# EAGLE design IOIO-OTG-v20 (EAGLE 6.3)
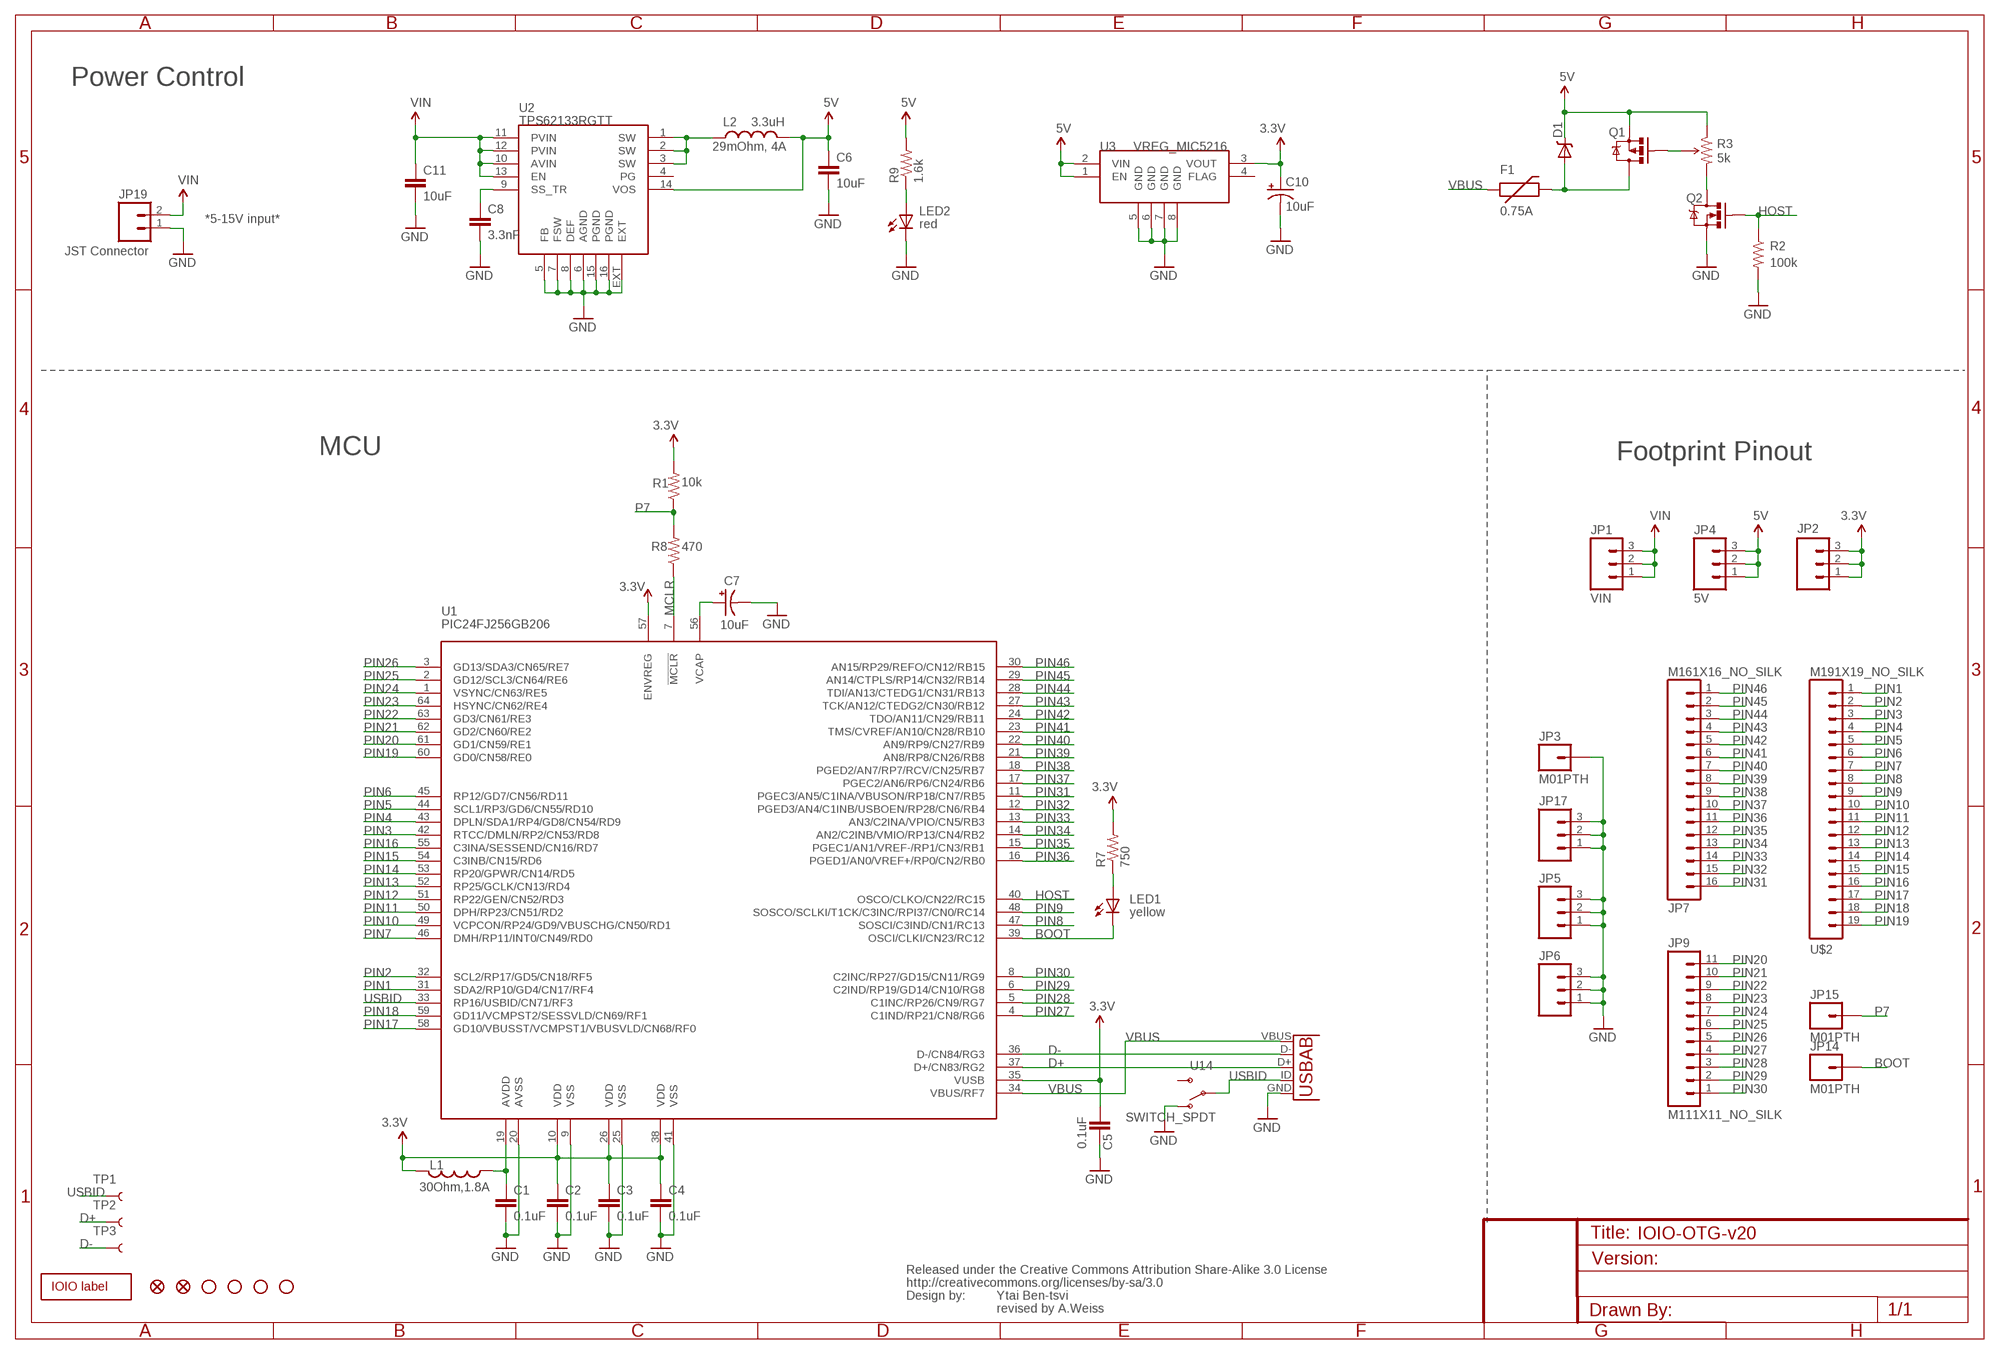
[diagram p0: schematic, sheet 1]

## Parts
C1  0.1uF  CAP0402-CAP  [0402-CAP]
C2  0.1uF  CAP0402-CAP  [0402-CAP]
C3  0.1uF  CAP0402-CAP  [0402-CAP]
C4  0.1uF  CAP0402-CAP  [0402-CAP]
C5  0.1uF  CAP0402-CAP  [0402-CAP]
C6  10uF  CAP0805  [0805]
C7  10uF  CAP_POL1206  [EIA3216]
C8  3.3nF  CAP0402-CAP  [0402-CAP]
C10  10uF  CAP_POL1206  [EIA3216]
C11  10uF  CAP1210  [1210]
D1  B340A  DIODE-SCHOTTKY_  [SMA-DIODE]
F1  PTCSMD  [PTC-1206]
JP1  VIN  M03PTH  [1X03]
JP2  M03PTH  [1X03]
JP3  M01PTH  [1X01]
JP4  5V  M03PTH  [1X03]
JP5  M03PTH  [1X03]
JP6  M03PTH  [1X03]
JP7  M161X16_NO_SILK  [1X16_NO_SILK]
JP8  FIDUCIALUFIDUCIAL  [MICRO-FIDUCIAL]
JP9  M111X11_NO_SILK  [1X11_NO_SILK]
JP10  STAND-OFF  [STAND-OFF]
JP11  STAND-OFF  [STAND-OFF]
JP12  STAND-OFF  [STAND-OFF]
JP13  STAND-OFF  [STAND-OFF]
JP14  M01PTH  [1X01]
JP15  M01PTH  [1X01]
JP16  FIDUCIALUFIDUCIAL  [MICRO-FIDUCIAL]
JP17  M03PTH  [1X03]
JP19  JST Connector  M02-JST-2MM-SMT  [JST-2-SMD]
L1  30Ohm,1.8A  INDUCTOR0402  [C0402]
L2  VLC5045T-3R3N  INDUCTORCR54  [CR54]
LED1  LY L29K-J1K2-26-Z  LED0603  [LED-0603]
LED2  LS L29K-G1J2-1-Z  LED0603  [LED-0603]
Q1  IRLML2244  MOSFET-PCHANNELSMD  [SOT23-3]
Q2  2N7002PW  MOSFET-NCHANNELSOT323  [SOT323]
R1  10k  RESISTOR0402-RES  [0402-RES]
R2  100k  RESISTOR0402-RES  [0402-RES]
R3  TS53YL502MR10  TRIMPOTTRIMPOT-5MM  [TRIMPOT-5MM]
R7  750  RESISTOR0402-RES  [0402-RES]
R8  470  RESISTOR0402-RES  [0402-RES]
R9  1.6k  RESISTOR0402-RES  [0402-RES]
TP1  TEST-POINT3  [PAD.03X.03]
TP2  TEST-POINT3  [PAD.03X.03]
TP3  TEST-POINT3  [PAD.03X.03]
U1  PIC24FJ256GB206  PIC24FXXXDAX06  [PIC24FXXX_TQFP64]
U2  TPS62133RGTT  TPS6214X  [QFN16-3X3MM]
U3  VREG_MIC5216  [MSOP8]
U14  SWITCH_SPDT  [KPS-1290]
U$1  CREATIVE_COMMONS  [CREATIVE_COMMONS]
U$2  M191X19_NO_SILK  [1X19_NO_SILK]
U$3  10104111-0001LF  USB_AB  [USB-AB-MICRO-SMD]
U$6  IOIO-OTG  [IOIO-OTG-COPPER-EXPOSED]

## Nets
3.3V: C2.1 C3.1 C4.1 C5.1 C10.A(+) JP2.1 JP2.2 JP2.3 L1.2 R1.2 R7.2 U1.10(VDD) U1.26(VDD) U1.35(VUSB) U1.38(VDD) U1.57(ENVREG) U3.3(VOUT)
5V: C6.1 D1.C JP4.1 JP4.2 JP4.3 L2.P$2 Q1.2(S) R3.A(CCW) R9.2 U2.14(VOS) U3.1(EN) U3.2(VIN)
BOOT: JP14.1 LED1.C U1.39(OSCI/CLKI/CN23/RC12)
D+: TP2.P$1 U1.37(D+/CN83/RG2) U$3.D+
D-: TP3.P$1 U1.36(D-/CN84/RG3) U$3.D-
GND: C1.2 C2.2 C3.2 C4.2 C5.2 C6.2 C7.C(-) C8.2 C10.C(-) C11.2 JP3.1 JP5.1 JP5.2 JP5.3 JP6.1 JP6.2 JP6.3 JP17.1 JP17.2 JP17.3 JP19.1 LED2.C Q2.2(S) R2.2 U1.9(VSS) U1.20(AVSS) U1.25(VSS) U1.41(VSS) U2.5(FB) U2.6(AGND) U2.7(FSW) U2.8(DEF) U2.15(PGND) U2.16(PGND) U2.EXT U3.5(GND) U3.6(GND) U3.7(GND) U3.8(GND) U14.O U$3.GND
HOST: Q2.1(G) R2.1 U1.40(OSCO/CLKO/CN22/RC15)
MCLR: R8.1 U1.7(!MCLR)
N$1: Q1.1(G) R3.B(WIPER)
N$2: LED1.A R7.1
N$3: LED2.A R9.1
N$4: D1.A F1.2 Q1.3(D)
N$5: C7.A(+) U1.56(VCAP)
N$6: L2.P$1 U2.1(SW) U2.2(SW) U2.3(SW)
N$7: C8.1 U2.9(SS_TR)
N$8: Q2.3(D) R3.C(CW)
N$9: C1.1 L1.1 U1.19(AVDD)
P7: JP15.1 R1.1 R8.2
PIN1: U1.31(SDA2/RP10/GD4/CN17/RF4) U$2.1
PIN2: U1.32(SCL2/RP17/GD5/CN18/RF5) U$2.2
PIN3: U1.42(RTCC/DMLN/RP2/CN53/RD8) U$2.3
PIN4: U1.43(DPLN/SDA1/RP4/GD8/CN54/RD9) U$2.4
PIN5: U1.44(SCL1/RP3/GD6/CN55/RD10) U$2.5
PIN6: U1.45(RP12/GD7/CN56/RD11) U$2.6
PIN7: U1.46(DMH/RP11/INT0/CN49/RD0) U$2.7
PIN8: U1.47(SOSCI/C3IND/CN1/RC13) U$2.8
PIN9: U1.48(SOSCO/SCLKI/T1CK/C3INC/RPI37/CN0/RC14) U$2.9
PIN10: U1.49(VCPCON/RP24/GD9/VBUSCHG/CN50/RD1) U$2.10
PIN11: U1.50(DPH/RP23/CN51/RD2) U$2.11
PIN12: U1.51(RP22/GEN/CN52/RD3) U$2.12
PIN13: U1.52(RP25/GCLK/CN13/RD4) U$2.13
PIN14: U1.53(RP20/GPWR/CN14/RD5) U$2.14
PIN15: U1.54(C3INB/CN15/RD6) U$2.15
PIN16: U1.55(C3INA/SESSEND/CN16/RD7) U$2.16
PIN17: U1.58(GD10/VBUSST/VCMPST1/VBUSVLD/CN68/RF0) U$2.17
PIN18: U1.59(GD11/VCMPST2/SESSVLD/CN69/RF1) U$2.18
PIN19: U1.60(GD0/CN58/RE0) U$2.19
PIN20: JP9.11 U1.61(GD1/CN59/RE1)
PIN21: JP9.10 U1.62(GD2/CN60/RE2)
PIN22: JP9.9 U1.63(GD3/CN61/RE3)
PIN23: JP9.8 U1.64(HSYNC/CN62/RE4)
PIN24: JP9.7 U1.1(VSYNC/CN63/RE5)
PIN25: JP9.6 U1.2(GD12/SCL3/CN64/RE6)
PIN26: JP9.5 U1.3(GD13/SDA3/CN65/RE7)
PIN27: JP9.4 U1.4(C1IND/RP21/CN8/RG6)
PIN28: JP9.3 U1.5(C1INC/RP26/CN9/RG7)
PIN29: JP9.2 U1.6(C2IND/RP19/GD14/CN10/RG8)
PIN30: JP9.1 U1.8(C2INC/RP27/GD15/CN11/RG9)
PIN31: JP7.16 U1.11(PGEC3/AN5/C1INA/VBUSON/RP18/CN7/RB5)
PIN32: JP7.15 U1.12(PGED3/AN4/C1INB/USBOEN/RP28/CN6/RB4)
PIN33: JP7.14 U1.13(AN3/C2INA/VPIO/CN5/RB3)
PIN34: JP7.13 U1.14(AN2/C2INB/VMIO/RP13/CN4/RB2)
PIN35: JP7.12 U1.15(PGEC1/AN1/VREF-/RP1/CN3/RB1)
PIN36: JP7.11 U1.16(PGED1/AN0/VREF+/RP0/CN2/RB0)
PIN37: JP7.10 U1.17(PGEC2/AN6/RP6/CN24/RB6)
PIN38: JP7.9 U1.18(PGED2/AN7/RP7/RCV/CN25/RB7)
PIN39: JP7.8 U1.21(AN8/RP8/CN26/RB8)
PIN40: JP7.7 U1.22(AN9/RP9/CN27/RB9)
PIN41: JP7.6 U1.23(TMS/CVREF/AN10/CN28/RB10)
PIN42: JP7.5 U1.24(TDO/AN11/CN29/RB11)
PIN43: JP7.4 U1.27(TCK/AN12/CTEDG2/CN30/RB12)
PIN44: JP7.3 U1.28(TDI/AN13/CTEDG1/CN31/RB13)
PIN45: JP7.2 U1.29(AN14/CTPLS/RP14/CN32/RB14)
PIN46: JP7.1 U1.30(AN15/RP29/REFO/CN12/RB15)
USBID: TP1.P$1 U1.33(RP16/USBID/CN71/RF3) U14.P U$3.ID(USBID)
VBUS: F1.1 U1.34(VBUS/RF7) U$3.VBUS
VIN: C11.1 JP1.1 JP1.2 JP1.3 JP19.2 U2.10(AVIN) U2.11(PVIN) U2.12(PVIN) U2.13(EN)
Unconnected: U2.4(PG) U3.4(FLAG) U14.S

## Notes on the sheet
- Power Control
- 29mOhm, 4A
- 5k
- 0.75A
- *5-15V input*
- red
- MCU | Footprint Pinout
- yellow
- Ytai Ben-tsvi
- revised by A.Weiss

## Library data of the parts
C1-C5 C8 = SparkFun:CAP: Capacitor
C6 = SparkFun-Passives:CAP: Capacitor; PART#: LMK212BJ106KG-T
C7 = SparkFun:CAP_POL: Capacitor Polarized
C10 = SparkFun-Passives:CAP_POL: Capacitor Polarized; PART#: TAJA106K016RNJ
C11 = SparkFun-Passives:CAP: Capacitor; PART#: UMK325C7106MM-T
D1 = SparkFun-DiscreteSemi:DIODE-SCHOTTKY: Commonly MBRA140.; PART#: B340A
F1 = SparkFun-PowerIC:PTC: Resettable Fuse PTC; PART#: 0ZCA0075FF2G
JP1 JP2 JP4-JP6 JP17 = SparkFun:M03: Header 3 Standard 3-pin 0.1" header. Use with straight break away headers (SKU : PRT-00116), right angle break away headers (PRT-00553), swiss pins (PRT-00743), machine pins (PRT-00117), and female headers (PRT-00115). Molex polarized connector foot print use with SKU : PRT-08232 with associated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
JP3 JP14 JP15 = SparkFun:M01: Header 1
JP7 = SparkFun-Connectors:M16: 1x16 .1" header
JP8 JP16 = SparkFun:FIDUCIAL: Fiducial Alignment Points
JP9 = SparkFun-Connectors:M11: Header 11 Standard 11-pin 0.1" header. Use with straight break away headers (SKU : PRT-00116), right angle break away headers (PRT-00553), swiss pins (PRT-00743), machine pins (PRT-00117), and female headers (PRT-00115).
JP10-JP13 = SparkFun:STAND-OFF: Stand Off
JP19 = SparkFun:M02: Header 2
L1 = SparkFun-Passives:INDUCTOR: Inductors
L2 = SparkFun-Passives:INDUCTOR: Inductors; AM: 3.3uH
LED1 LED2 = SparkFun:LED: LEDs
Q1 = SparkFun-DiscreteSemi:MOSFET-PCHANNEL: Generic PMOSFET
Q2 = SparkFun-DiscreteSemi:MOSFET-NCHANNEL: Generic NMOS footprint; PART#: 2N7002PW
R1 R2 R7-R9 = SparkFun:RESISTOR: Resistor
R3 = SparkFun-Electromechanical:TRIMPOT: Various small potentiometers for "set-and-forget" applications; PART#: TS53YL502MR10
TP1-TP3 = SparkFun-Passives:TEST-POINT: Bare copper test points for troubleshooting or ICT
U1 = SparkFun-DigitalIC:PIC24FXXXDAX06: PIC24FXXXDAX06 PIC24FXXXDA106 / PIC24FXXXDA206
U2 = SparkFun-PowerIC:TPS6214X: 3-17V, 2A Step Down Converter
U3 = SparkFun-PowerIC:VREG_MIC5216: 500mA LDO, MSOP8 for better dissipation
U14 = SparkFun-Electromechanical:SWITCH_SPDT: Side-actuated SPDT slide switch, as used on the Arduino Pro
U$1 = SparkFun-Aesthetics:CREATIVE_COMMONS: Creative Commons License summary
U$2 = SparkFun-Connectors:M19: 1x19 .1" header
U$3 = SparkFun-Connectors:USB_AB: This is a USB AB connector that is compatible with USB OTG. i.e. this connector can serve as a host or device
U$6 = SparkFun-Aesthetics:IOIO-OTG: Labels for the IOIO-OTG

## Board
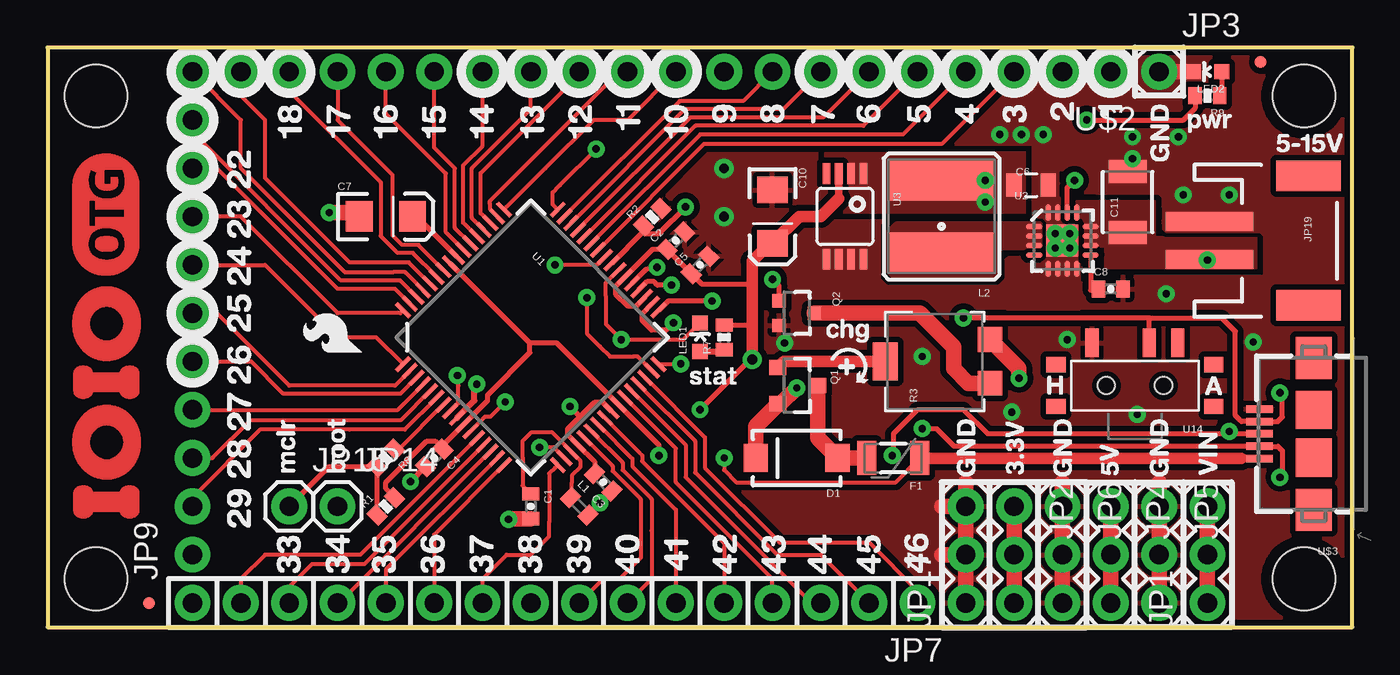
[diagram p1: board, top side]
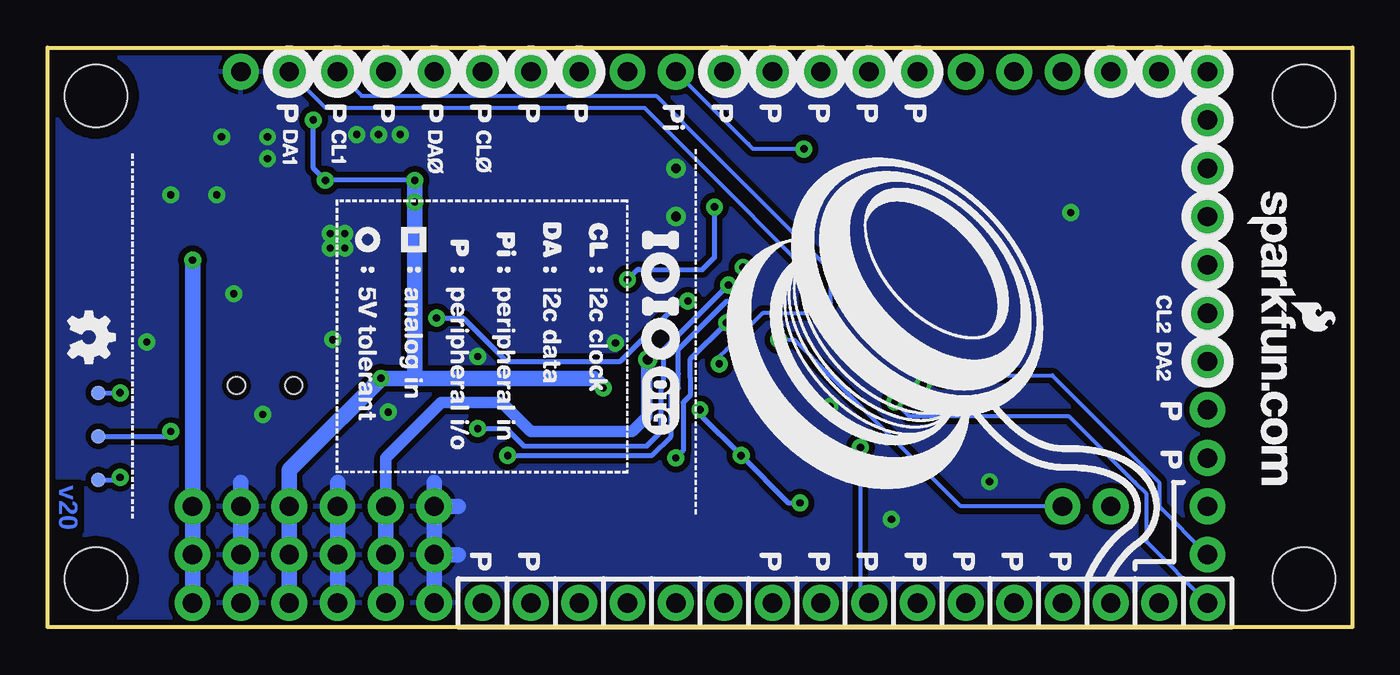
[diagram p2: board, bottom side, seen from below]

Size 68.58 x 30.48 mm. Coordinates in mm from the lower left corner, seen from the top.
Outline: 0,0 68.58,0 68.58,30.48 0,30.48 0,0
Copper layers (1*16): Top 0.035mm / dielectric 1.5mm / Bottom 0.035mm
Design rules "default": minimum track width 8mil, minimum drill 15mil, track to track 8mil, track to pad 8mil, pad to pad 8mil, via to via 8mil, smd to smd 8mil, copper to edge 8mil, drill to drill 8mil, minimum pad ring 12mil, minimum via ring 10mil, stop-mask expansion 4mil, vias tented up to drill 20mil, thermal gap 10mil

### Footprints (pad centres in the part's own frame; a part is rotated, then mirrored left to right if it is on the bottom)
0402-CAP = smd 0.7 x 0.9: 1 -0.65,0; 2 0.65,0
0805 = smd 0.8 x 1.2: 1 -0.9,0; 2 0.9,0
EIA3216 = smd 1.4 x 1.6: A 1.4,0; C -1.4,0
1210 = smd 1.2 x 2: 1 -1.6,0; 2 1.6,0
SMA-DIODE = smd 1.27 x 1.47: A -2.15,0; C 2.15,0
PTC-1206 = smd 1 x 1.8: 1 -1.4,0; 2 1.4,0
1X03 = drill 1.016 pad 1.88: 1 0,0; 2 2.54,0; 3 5.08,0
1X01 = drill 1.016 pad 1.88: 1 0,0
1X16_NO_SILK = drill 1.016 pad 1.88: 1 0,0; 2 2.54,0; 3 5.08,0; 4 7.62,0; 5 10.16,0; 6 12.7,0; 7 15.24,0; 8 17.78,0; 9 20.32,0; 10 22.86,0; 11 25.4,0; 12 27.94,0; 13 30.48,0; 14 33.02,0; 15 35.56,0; 16 38.1,0
MICRO-FIDUCIAL = smd 0.635 x 0.635: 1 0,0
1X11_NO_SILK = drill 1.016 pad 1.88: 1 0,0; 2 2.54,0; 3 5.08,0; 4 7.62,0; 5 10.16,0; 6 12.7,0; 7 15.24,0; 8 17.78,0; 9 20.32,0; 10 22.86,0; 11 25.4,0
STAND-OFF = hole 3.302: 0,0
JST-2-SMD = smd 1 x 4.6: 1 -1,-3.7; 2 1,-3.7 | smd 1.6 x 3.4: NC1 -3.4,1.5; NC2 3.4,1.5
C0402 = smd 0.7 x 0.9: 1 -0.65,0; 2 0.65,0
CR54 = smd 5.5 x 2.15: P$1 0,1.92; P$2 0,-1.92
LED-0603 = smd 0.8 x 0.8: A 0,-0.75; C 0,0.75
SOT23-3 = smd 0.8 x 0.9: 1 -0.95,-1; 2 0.95,-1; 3 0,1.1
SOT323 = smd 0.7 x 0.7: 1 -0.65,-0.925; 2 0.65,-0.925; 3 0,0.925
0402-RES = smd 0.7 x 0.9: 1 -0.65,0; 2 0.65,0
TRIMPOT-5MM = smd 1.3 x 1.3: A 1.15,-2.54; C -1.15,-2.54 | smd 2 x 1.3: B 0,2.96
PAD.03X.03 = smd 0.762 x 0.762: P$1 0,0
PIC24FXXX_TQFP64 = smd 0.22 x 1: 1 -3.75,-5.75; 2 -3.25,-5.75; 3 -2.75,-5.75; 4 -2.25,-5.75; 5 -1.75,-5.75; 6 -1.25,-5.75; 7 -0.75,-5.75; 8 -0.25,-5.75; 9 0.25,-5.75; 10 0.75,-5.75; 11 1.25,-5.75; 12 1.75,-5.75; 13 2.25,-5.75; 14 2.75,-5.75; 15 3.25,-5.75; 16 3.75,-5.75; 33 3.75,5.75; 34 3.25,5.75; 35 2.75,5.75; 36 2.25,5.75; 37 1.75,5.75; 38 1.25,5.75; 39 0.75,5.75; 40 0.25,5.75; 41 -0.25,5.75; 42 -0.75,5.75; 43 -1.25,5.75; 44 -1.75,5.75; 45 -2.25,5.75; 46 -2.75,5.75; 47 -3.25,5.75; 48 -3.75,5.75 | smd 1 x 0.22: 17 5.75,-3.75; 18 5.75,-3.25; 19 5.75,-2.75; 20 5.75,-2.25; 21 5.75,-1.75; 22 5.75,-1.25; 23 5.75,-0.75; 24 5.75,-0.25; 25 5.75,0.25; 26 5.75,0.75; 27 5.75,1.25; 28 5.75,1.75; 29 5.75,2.25; 30 5.75,2.75; 31 5.75,3.25; 32 5.75,3.75; 49 -5.75,3.75; 50 -5.75,3.25; 51 -5.75,2.75; 52 -5.75,2.25; 53 -5.75,1.75; 54 -5.75,1.25; 55 -5.75,0.75; 56 -5.75,0.25; 57 -5.75,-0.25; 58 -5.75,-0.75; 59 -5.75,-1.25; 60 -5.75,-1.75; 61 -5.75,-2.25; 62 -5.75,-2.75; 63 -5.75,-3.25; 64 -5.75,-3.75
QFN16-3X3MM = smd 0.85 x 0.28: 1 -1.475,0.75; 2 -1.475,0.25; 3 -1.475,-0.25; 4 -1.475,-0.75; 9 1.475,-0.75; 10 1.475,-0.25; 11 1.475,0.25; 12 1.475,0.75 | smd 0.28 x 0.85: 5 -0.75,-1.475; 6 -0.25,-1.475; 7 0.25,-1.475; 8 0.75,-1.475; 13 0.75,1.475; 14 0.25,1.475; 15 -0.25,1.475; 16 -0.75,1.475 | smd 1.68 x 1.68: EXT 0,0
MSOP8 = smd 0.4 x 1.1: 1 -0.975,-2.25; 2 -0.325,-2.25; 3 0.325,-2.25; 4 0.975,-2.25; 5 0.975,2.25; 6 0.325,2.25; 7 -0.325,2.25; 8 -0.975,2.25
KPS-1290 = smd 0.7 x 1.5: O -2.25,2.25; P 0.75,2.25; S 2.25,2.25 | smd 1 x 0.8: P$1 -4.15,1.1; P$2 -4.15,-1.1; P$3 4.15,-1.1; P$4 4.15,1.1 | hole 0.9: -1.5,0; 1.5,0
1X19_NO_SILK = drill 1.016 pad 1.88: 1 0,0; 2 2.54,0; 3 5.08,0; 4 7.62,0; 5 10.16,0; 6 12.7,0; 7 15.24,0; 8 17.78,0; 9 20.32,0; 10 22.86,0; 11 25.4,0; 12 27.94,0; 13 30.48,0; 14 33.02,0; 15 35.56,0; 16 38.1,0; 17 40.64,0; 18 43.18,0; 19 45.72,0
USB-AB-MICRO-SMD = smd 1.4 x 0.4: D+ 2.85,0; D- 2.85,0.65; GND 2.85,-1.3; ID 2.85,-0.65; VBUS 2.85,1.3 | smd 1.9 x 2: P$6 0,1.25; P$7 0,-1.25 | smd 1.9 x 2.2: P$8 0,4; P$9 0,-4

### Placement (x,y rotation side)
C1  25.4,6.35 270 top
C2  33.02,20.32 45 top
C3  29.21,7.62 135 top
C4  20.32,8.89 225 top
C5  34.29,19.05 45 top
C6  51.69,23.24 0 top
C7  17.78,21.59 0 top
C8  55.88,17.78 0 top
C10  38.1,21.59 270 top
C11  56.77,22.35 90 top
D1  39.37,8.89 180 top
F1  44.45,8.89 180 top
JP1  60.96,1.27 90 top
JP2  50.8,6.35 270 top
JP3  58.42,29.21 0 top
JP4  55.88,6.35 270 top
JP5  58.42,6.35 270 top
JP6  53.34,6.35 270 top
JP7  45.72,1.27 180 top
JP8  5.33,1.27 0 top
JP9  7.62,3.81 90 top
JP10  66.04,27.94 0 top
JP11  66.04,2.54 0 top
JP12  2.54,27.94 0 top
JP13  2.54,2.54 0 top
JP14  15.24,6.35 0 top
JP15  12.7,6.35 0 top
JP16  63.75,29.72 0 top
JP17  48.26,1.27 90 top
JP19  64.77,20.32 270 top
L1  27.94,6.35 315 top
L2  46.99,21.59 180 top
LED1  34.29,15.24 0 top
LED2  60.96,29.21 90 top
Q1  39.37,12.7 270 top
Q2  39.37,16.51 270 top
R1  17.78,6.35 45 top
R2  31.78,21.56 45 top
R3  46.99,13.97 90 top
R7  35.56,15.24 90 top
R8  17.78,8.89 225 top
R9  60.96,27.94 180 top
TP1  65.91,12.32 0 bottom
TP2  65.91,10.03 0 bottom
TP3  65.91,7.75 0 bottom
U1  25.4,15.24 315 top
U2  53.34,20.32 0 top
U3  41.91,21.59 180 top
U14  57.15,12.7 0 top
U$1  not placed on the board
U$2  55.88,29.21 180 top
U$3  66.55,10.16 180 top
U$6  4.83,5.71 90 top

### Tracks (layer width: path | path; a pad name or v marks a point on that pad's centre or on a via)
3.3V  (via drill 0.38, 0.51)
  Top 0.203: U1.38 | 20.78,9.37 C4.1
  Top 0.254: U1.38 31.79,19.86 C2.1 C5.1 34.39,18.03 36.78,18.03 37.03,17.78 | U1.38 29.84,17.92 29.84,17.53 30.48,16.89 30.94,16.89 U1.35 | v32.13,9.02 32.13,9.57 U1.26 26.76,14.94 25.35,14.94 | L1.2 v29.03,6.52 v29.03,6.53 v29.04,6.53 C3.1 | 20.78,9.56 U1.10 23.11,11.89 23.11,12.19 25.35,14.43 25.35,14.94 | R1.2 17.78,7.27 17.78,7.62 19.94,9.78 20.37,9.78 20.78,9.37 | 25.35,14.94 U1.57 | R7.2 37.02,15.89 37.03,15.88 | v34.29,11.43 36.93,14.07 v37.03,14.07 | 38.1,20.32 C10.A
  Top 0.305: 20.78,9.56 C4.1
  Top 0.406: U3.3 41.59,22.54
  Top 0.61: v37.03,14.07 37.03,15.88 37.03,17.78 37.03,19.25 38.1,20.32 | 41.59,22.54 40.64,21.59 39.5,21.59 C10.A
  Top 0.813: JP2.1 JP2.2 JP2.3
  Bottom 0.254: v34.29,11.43 34.29,11.18 v32.13,9.02 29.64,6.53 v29.03,6.53
  Bottom 0.61: JP2.1 50.8,8.89 47.88,11.81 44.7,11.81 43.18,10.29 37.85,10.29 37.08,11.05 37.08,14.02 v37.03,14.07
  Bottom 0.813: JP2.3 JP2.1
5V  (via drill 0.38)
  Top 0.254: U2.14 53.59,23.11 v53.98,23.5 | R9.2 60.31,27.29 59.69,26.67 v54.61,26.67
  Top 0.813: JP4.1 JP4.2 JP4.3 | R3.A 49.53,15.24 | Q1.2 38.42,11.75 | R3.A | D1.C 37.22,10.55 38.42,11.75 | R3.A | R3.A 51.05,13.59 v51.05,13.08 | 38.42,11.75 38.55,11.75 v39.37,12.57
  Bottom 0.254: v53.98,23.5 54.61,24.13 | 54.61,24.13 v54.61,26.67 | v49.28,23.5 53.85,23.5 v53.98,23.5 | v53.98,23.5 54.61,24.13
  Bottom 0.813: JP4.3 JP4.1 55.88,7.62 55.88,8.26 55.24,8.89 v51.05,13.08 49.53,13.08 | 49.53,13.08 40.39,13.08 39.88,13.08 v39.37,12.57 | v49.28,23.5 49.28,13.34 49.53,13.08
  other vias: 49.28,22.35
  pour Top (isolate 0.305, rank 2, no thermals): 40.89,21.84 51.56,21.84 51.56,24.89 40.89,24.89
BOOT  (via drill 0.38)
  Top 0.203: U1.39 29.34,18.12 29.34,17.4 29.34,17.02 29.34,15.93 v30.15,15.11 33.41,15.11 LED1.C
  Top 0.254: LED1.C 34.28,15.99
  Bottom 0.203: JP14.1 20.32,6.35 20.57,6.35 28.19,13.97 | 28.19,13.97 28.45,14.22 | 28.19,13.97 28.45,14.22 | v30.15,15.11 29.34,15.11 28.45,14.22
D+  (via drill 0.38)
  Top 0.254: v32.03,18.92 31.43,18.8 U1.37 | v62.1,10.29 62.23,10.16 U$3.D+ 49.4,10.16 48.13,11.43 45.72,11.43 44.45,10.16 44.45,9.07 v44.4,9.02
  Bottom 0.254: v32.03,18.92 32,18.9 32,17.65 32.51,17.14 32.89,17.14 35.43,14.61 35.43,13.34 35.43,12.57 35.81,12.19 35.81,10.03 36.83,9.02 39.24,9.02 v44.4,9.02 | TP2.P$1 62.36,10.03 v62.1,10.29
D-  (via drill 0.38)
  Top 0.254: v32.79,17.98 32.05,17.98 31.88,18.16 31.5,18.16 U1.36 | v64.77,7.87 64.9,8 64.9,9.27 64.66,9.51 U$3.D- 48.4,9.51 47.64,9.51 46.99,10.16 46.71,10.44 v45.97,10.44
  Bottom 0.254: v32.79,17.98 32.82,17.98 36.2,14.61 36.2,13.46 36.2,12.7 36.32,12.57 36.32,10.29 37.08,9.53 43.56,9.53 44.48,10.44 v45.97,10.44 | TP3.P$1 64.9,7.75 v64.77,7.87
GND  (via drill 0.38, 0.38 pad 0.03, 0.51)
  Top 0.203: 24.39,5.7 v24.23,5.66 | U1.41 28.86,19.05 v26.67,19.05
  Top 0.254: C3.2 28.75,8.71 U1.20 27.33,10.13 27.33,10.41 28,11.09 | U1.25 29.18,11.81 28.73,11.81 28,11.09 | C7.C 16.18,21.79 | v27.46,11.61 27.98,11.09 28,11.09
  Top 0.305: U1.9 22.43,11.91 22.43,12.65 v22.55,12.78 | C4.2 v19.07,7.64
  Top 0.813: 16.18,21.79 v14.81,21.79 | C1.2 24.39,5.7 | JP6.3 53.34,7.62 | JP17.1 JP17.2 | JP17.2 JP17.3 | JP17.3 48.26,7.62 | JP17.3 46.99,6.35 | JP17.2 46.99,3.81 | 58.42,7.62 JP5.3 | LED2.C JP3.1
  Bottom 0.813: 48.26,7.62 JP17.3 | JP17.3 JP17.2 | JP17.2 JP17.1 | JP17.3 46.99,6.35 | JP17.2 46.99,3.81 | 53.34,7.62 JP6.3 | 58.42,7.62 JP5.3
  other vias: 59.69,22.73 62.1,22.73 58.8,17.53 63.37,14.99 57.28,11.18 45.97,14.22 38.73,14.94 52.96,20.7 53.72,20.7 52.96,19.94 53.72,19.94 50.67,11.3 53.59,15.11 59.44,25.78 57.02,25.78 57.02,24.64 52.32,25.91 51.18,25.91 50.04,25.91 35.56,24.13 35.56,21.59
  pour Bottom (isolate 0.305): 6.35,30.48 68.58,30.48 68.58,0 6.35,0
  pour Top (isolate 0.305, rank 6): 32.03,30.35 32.03,-0.13 68.58,0 68.58,30.48
  pour Top (no thermals): 40.51,20.07 40.51,18.41 43.31,18.41 43.31,20.07
  pour Top (no thermals): 53.34,22.35 53.09,22.61 53.09,25.02 52.96,25.15 52.07,25.15 51.82,24.89 51.82,21.84 52.07,21.59 52.32,21.59 52.58,21.34 52.58,19.43 52.2,19.05 50.55,19.05 50.42,18.92 50.42,16.76 54.23,16.76 54.23,19.05 54.1,19.18 54.1,21.08 53.34,21.08
  pour Top (isolate 0.305, no thermals): 68.58,19.05 68.58,30.48 51.82,30.48 51.82,24.13 54.36,24.13 54.86,23.62 54.86,23.11 55.12,22.86 58.42,22.86 58.67,22.61 58.67,20.95 58.8,20.83 63.75,20.83 64.01,20.57 64.01,18.92 68.45,18.92
HOST  (via drill 0.38)
  Top 0.254: R2.1 31.29,20.78 | 31.29,20.78 U1.40 | v33.53,22.1 32.13,20.7 31.37,20.7 31.29,20.78 | Q2.1 38.45,17.82 38.45,17.94 v38.1,18.29
  Bottom 0.254: v33.53,22.1 33.53,19.43 34.16,18.8 37.47,18.8 37.59,18.8 v38.1,18.29
MCLR
  Top 0.203: U1.7 18.45,9.35 R8.1
N$1
  Top 0.61: R3.B 38.69,13.97 Q1.1
N$2
  Top 0.305: LED1.A 35.46,14.49 R7.1
N$3
  Top 0.254: LED2.A 61.71,28.04 R9.1
N$4
  Top 0.813: F1.2 D1.A 40.47,9.94 Q1.3
N$5
  Top 0.203: 19.4,21.59 C7.A
  Top 0.254: U1.56 19.4,21.59
N$6
  pour Top (no thermals): 52.2,20.07 52.2,21.21 44.58,21.21 44.2,20.83 44.2,18.67 44.45,18.41 49.66,18.41 49.91,18.67 49.91,19.68 50.16,19.94 52.07,19.94
N$7
  Top 0.254: U2.9 54.81,17.72 C8.1
N$8
  Top 0.813: R3.C 48.39,12.82 47.62,13.59 47.62,14.73 45.85,16.51 Q2.3
N$9
  Top 0.203: C1.1 24.97,7.43 24.97,8.91 24.97,9.78 25.45,10.26 26.49,10.26 26.97,9.78 U1.19 27.99,8.76 27.99,8.41 27.56,7.98 27.56,7.62 27.56,6.89 L1.1
P7
  Top 0.254: JP15.1 14.78,8.43 R8.2 R1.1
PIN1  (via drill 0.38)
  Top 0.203: v28.35,17.32 28.35,16.89 28.35,16.48 28.35,15.44 29.03,14.76 29.57,14.22 30.76,14.22 31.01,14.22 U1.31
  Bottom 0.203: v28.35,17.32 28.35,18.44 28.91,19 34.04,24.13 37.21,27.3 53.98,27.3 U$2.1
PIN2  (via drill 0.38)
  Top 0.203: U1.32 32.13,13.84 v33.27,13.84
  Bottom 0.203: v33.27,13.84 33.27,14.22 32.89,14.61 30.99,16.51 30.48,16.51 27.94,16.51 27.41,17.04 27.41,18.75 33.81,25.15 36.6,27.94 52.07,27.94 U$2.2
PIN3
  Top 0.203: U$2.3 46.99,25.4 34.5,25.4 U1.42
PIN4
  Top 0.203: U$2.4 44.96,25.91 34.3,25.91 U1.43
PIN5
  Top 0.203: U$2.5 42.88,26.36 34.05,26.36 U1.44
PIN6
  Top 0.203: U$2.6 40.77,26.8 33.77,26.8 U1.45
PIN7
  Top 0.203: U$2.7 38.66,27.23 33.5,27.23 U1.46
PIN8
  Top 0.203: U$2.8 36.55,27.66 33.22,27.66 U1.47
PIN9  (via drill 0.38)
  Top 0.203: v28.83,25.15 26.92,23.24 26.54,22.86 26.54,22.23 U1.48
  Bottom 0.203: U$2.9 31.75,25.4 31.5,25.15 v28.83,25.15
PIN10
  Top 0.203: U1.49 26.16,24.13 28.7,26.67 30.48,26.67 U$2.10
PIN11
  Top 0.203: U1.50 23.24,22 23.24,22.25 23.24,22.4 29.39,28.55 30.05,29.21 U$2.11
PIN12
  Top 0.203: U1.51 22.76,21.77 22.76,22.15 22.76,23.88 27.43,28.55 27.94,29.06 U$2.12
PIN13
  Top 0.203: U1.52 22.3,21.52 22.3,24.13 25.4,27.23 U$2.13
PIN14
  Top 0.203: U1.53 21.84,21.27 21.84,24.13 21.84,24.28 22.86,25.3 U$2.14
PIN15
  Top 0.203: U1.54 21.41,21 21.41,24.13 20.32,25.22 U$2.15
PIN16
  Top 0.203: U1.55 20.93,20.77 20.93,23.85 17.78,27 U$2.16
PIN17
  Top 0.203: U$2.17 15.24,26.67 17.78,24.13 18.14,23.77 18.14,20.6 18.21,20.52 18.64,20.09 19.49,20.09 U1.58
PIN18
  Top 0.203: U$2.18 12.7,28.19 17.5,23.39 17.5,20.57 18.4,19.67 19.2,19.67 U1.59
PIN19
  Top 0.203: U1.60 18.99,19.18 18.29,19.18 15.88,19.18 14.99,20.07 13.97,21.08 11.43,23.62 11.43,26.67 10.16,27.94 U$2.19
PIN20
  Top 0.203: U1.61 18.79,18.67 18.16,18.67 15.62,18.67 15.24,19.05 12.7,21.59 10.16,24.13 10.16,26.67 JP9.11
PIN21
  Top 0.203: U1.62 18.59,18.16 18.51,18.24 16.76,18.24 15.49,18.24 15.42,18.24 7.62,26.04 JP9.10
PIN22
  Top 0.203: U1.63 18.26,17.78 15.24,17.78 8.89,24.13 JP9.9
PIN23
  Top 0.203: U1.64 18.54,16.51 15.24,16.51 10.16,21.59 JP9.8
PIN24
  Top 0.203: U1.1 17.27,15.24 15.24,15.24 11.43,19.05 JP9.7
PIN25
  Top 0.203: U1.2 18.26,12.7 12.7,12.7 8.89,16.51 JP9.6
PIN26
  Top 0.203: U1.3 18.54,12.27 12.39,12.27 10.69,13.97 JP9.5
PIN27
  Top 0.203: U1.4 18.41,11.43 JP9.4
PIN28
  Top 0.203: U1.5 18.56,10.87 10.64,10.87 8.66,8.89 JP9.3
PIN29
  Top 0.203: U1.6 18.78,10.39 15.88,10.39 11.18,10.39 7.62,6.83 JP9.2
PIN30  (via drill 0.38)
  Top 0.203: U1.8 21.59,11.78 21.59,12.7 21.59,13.18 v21.54,13.23
  Bottom 0.203: v21.54,13.23 15.77,13.23 10.16,7.62 10.16,6.35 JP9.1
PIN31  (via drill 0.38)
  Top 0.203: U1.11 23,11.07 23.29,11.07 v24.05,11.84
  Bottom 0.203: JP7.16 10.85,4.5 10.85,7.04 11.43,7.62 14.88,11.07 23.29,11.07 v24.05,11.84
PIN32
  Top 0.203: U1.12 16.45,3.81 11.43,3.81 10.16,2.54 JP7.15
PIN33
  Top 0.203: U1.13 16.64,3.3 13.89,3.3 12.7,2.11 JP7.14
PIN34
  Top 0.203: U1.14 15.32,1.27 JP7.13
PIN35
  Top 0.203: U1.15 17.78,3.02 JP7.12
PIN36
  Top 0.203: U1.16 20.32,4.86 JP7.11
PIN37
  Top 0.203: JP7.10 22.86,2.54 24.13,3.81 25.4,3.81 26.36,4.78 26.36,5.51 26.36,8.07 26.67,8.38 U1.17
PIN38  (via drill 0.38)
  Top 0.203: U1.18 26.59,9.45 v25.86,9.45
  Bottom 0.203: v25.86,9.45 25.86,1.73 JP7.9
PIN39
  Top 0.203: U1.21 29.69,8.47 29.69,8.2 31.17,6.73 31.17,3.63 30.07,2.54 29.21,2.54 JP7.8
PIN40
  Top 0.203: U1.22 30.23,8.65 30.23,8.26 31.75,6.73 31.75,5.08 31.75,2.54 JP7.7
PIN41
  Top 0.203: U1.23 30.73,8.85 30.73,8.46 33.02,6.17 JP7.6
PIN42
  Top 0.203: U1.24 31.11,9.17 31.24,9.04 31.24,8.71 35.56,4.39 35.56,4.19 JP7.5
PIN43
  Top 0.203: JP7.4 38.1,2.54 33.02,7.62 33.02,9.39 U1.27
PIN44
  Top 0.203: U1.28 33.53,9.59 33.53,7.87 40.13,1.27 JP7.3
PIN45
  Top 0.203: U1.29 34.04,9.79 34.04,8.13 38.35,3.81 40.64,3.81 JP7.2
PIN46
  Top 0.203: U1.30 34.54,9.98 34.54,8.38 38.48,4.45 43.18,4.45 45.72,1.91 JP7.1
USBID  (via drill 0.38)
  Top 0.254: 57.91,16.26 61.72,16.26 62.43,15.54 62.43,11.12 62.61,10.95 62.75,10.81 U$3.ID 64.66,10.81 64.9,11.05 64.9,12.19 v64.77,12.32 | 57.91,16.26 v48.13,16.26 | U14.P 57.9,16.24 57.91,16.26 | v34.92,17.14 32.61,17.14 U1.33
  Bottom 0.254: v48.13,16.26 46.74,16.26 44.45,13.97 38.48,13.97 35.31,17.14 v34.92,17.14 | TP1.P$1 v64.77,12.32
VBUS  (via drill 0.38)
  Top 0.203: v35.56,8.89 35.56,8.26 36.2,7.62 44.58,7.62 F1.1 45.88,8.86
  Top 0.254: v32.89,16 32.51,15.62 31.75,15.62 31.24,16.13 31.24,16.49 U1.34
  Top 0.381: U$3.VBUS 62.74,8.86
  Top 0.61: 45.88,8.86 62.74,8.86
  Bottom 0.254: v32.89,16 34.8,14.1 34.8,13.08 34.8,12.19 35.05,11.94 35.18,11.81 35.18,9.27 v35.56,8.89
VIN  (via drill 0.38)
  Top 0.203: U2.11 U2.10
  Top 0.813: JP1.3 JP1.2 | JP1.2 JP1.1 JP1.2
  Bottom 0.813: JP1.1 JP1.3 v60.96,19.3
  pour Top (isolate 0.305, no thermals): 55.63,20.07 55.63,18.92 63.5,18.92 63.5,20.45 58.17,20.45 58.17,22.35 54.1,22.35 54.1,21.59 54.36,21.59 54.48,21.46 54.48,20.07

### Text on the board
Bottom: v20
